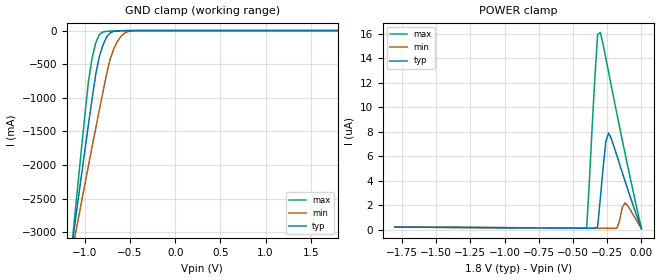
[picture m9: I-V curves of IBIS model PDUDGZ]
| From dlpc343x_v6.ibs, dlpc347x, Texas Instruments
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[Model]  PDUDGZ
Model_type Input
Polarity   Non-Inverting
Vinl =   0.6300V
Vinh =   1.1700V
C_comp   3.3702pF   3.2612pF   3.5114pF
[Temperature Range]   25.0000   0.1250k   -40.0000
[Voltage Range]   1.8000V   1.6200V   1.9800V
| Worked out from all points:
|   GND clamp passes 1 mA (typ) near -0.53 V on its own axis
[GND_clamp]
|Voltage   I(typ)   I(min)   I(max)
-1.8V     -9.929A    -8.053A    -12.56A
-1.16V    -3.375A    -3.424A    -3.437A
-1.12V    -2.974A    -3.138A    -2.882A
-1.08V    -2.574A    -2.854A    -2.333A
-960mV    -1.399A    -2.009A    -757.1mA
-920mV    -1.019A    -1.731A    -410.8mA
-880mV    -652.7mA   -1.455A    -184.5mA
-800mV    -215.1mA   -916mA     -20.61mA
-720mV    -33.92mA   -424.5mA   -7.988mA
-680mV    -11.51mA   -271.8mA   -5.699mA
-520mV    -753.8uA   -14.09mA   -653uA
1.8V      83.42nA    110.5nA    -8.113uA
[POWER_clamp]
|Voltage   I(typ)   I(min)   I(max)
-1.8V     208.3nA    217.7nA    217nA
-400mV    117nA      124.3nA    126.5nA
-340mV    113nA      120.3nA    12.45uA
-320mV    224.4nA    119nA      15.94uA
-300mV    2.565uA    117.6nA    16.13uA
-260mV    7.215uA    114.9nA    14.02uA
-240mV    7.9uA      113.6nA    12.88uA
-180mV    6.082uA    110.5nA    9.512uA
-160mV    5.374uA    700.9nA    8.411uA
-140mV    4.672uA    1.814uA    7.323uA
-120mV    3.979uA    2.186uA    6.248uA
0V        83.42nA    87.03nA    91.38nA
